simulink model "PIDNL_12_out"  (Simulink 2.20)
settings: Solver=VariableStepDiscrete  StartTime=0.0  StopTime=40.0  RelTol=1e-3  AbsTol=1e-6
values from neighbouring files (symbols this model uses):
  a = input('Inserisci il dato da graficare [1=PIDNL 2=PD 3=PID]: ')    [grp.m]    (also in grp1.m = input('Inserisci il dato da graficare [1..3]'))
undefined symbols (not defined in the file or in its folder): b, nldelta, pidin
libraries: simulink x3, Puma x2

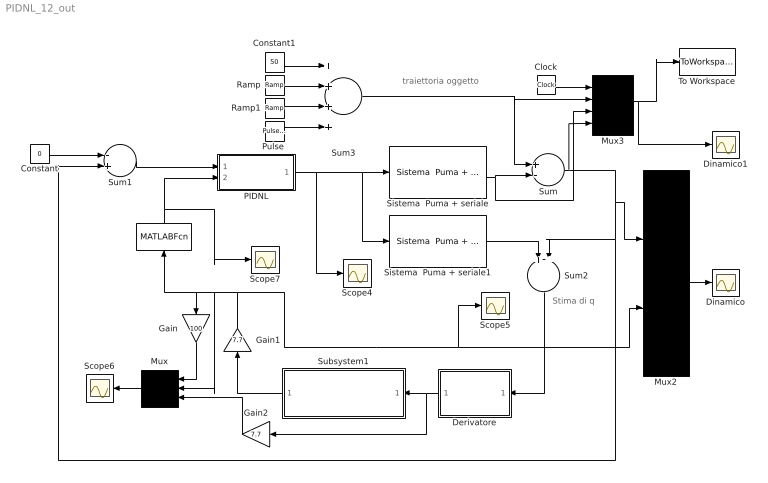
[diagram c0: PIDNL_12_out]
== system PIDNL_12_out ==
  note: Stima di q
  note: traiettoria oggetto
  " " : MATLABFcn  Orientation=up  MATLABFcn=nldelta(u(1))  OutputWidth=-1
  Clock : Clock
  Constant : Constant  Value=0
  Constant1 : Constant  Value=50
  Derivatore : Subsystem  Orientation=left  mask(Simulazione Derivatore implementato in maniera software){Td=0.13, T=0.030, N=5}
      mask prompts: Td "Costante di derivazione Td"; T "Sample Time T del PD"; N "Indice polo del derivatore [5..10]"
      mask init:
      | Kbeta=Td/(N*T+Td);
      | Kalfa=N*Kbeta;
  Dinamico : Scope
  Dinamico1 : Scope
  Gain : Gain  Orientation=down  Gain=100
  Gain1 : Gain  Orientation=up  Gain=7.7
  Gain2 : Gain  Orientation=left  Gain=7.7
  Mux : Mux  Orientation=left  Inputs=3
  Mux2 : Mux  Inputs=2
  Mux3 : Mux  Inputs=4
  PIDNL : Subsystem
  "Pulse " : simulink/Sources/Pulse Generator  period=30  duty=10  amplitude=-50  start=30
  Ramp : simulink/Sources/Ramp  slope=-50  start=10  X0=0
  Ramp1 : simulink/Sources/Ramp  slope=+50  start=25  X0=0
  Scope{4..7} (4 alike) : Scope
  Sistema  Puma + seriale : Puma/Sistema  Puma + seriale  Ts=.260
  Sistema  Puma + seriale1 : Puma/Sistema  Puma + seriale  Ts=.260
  Subsystem1 : Subsystem  Orientation=left  mask(Filtro di Butterworth){ordine=3, freq=0.1/16}
      mask prompts: ordine "Ordine del filtro"; freq "Parametro K per ricavare la Freq. di taglio Ft"
      mask help: Attenzione! Considerare il parametro Fc come la frequanza di campionamento del segnale di ingresso, per cui la frequanza di taglio diviene Ft=K*Fc;
      mask init:
      | [b,a]=butter(ordine,freq);
  Sum : Sum  Inputs=+-
  Sum1 : Sum  Inputs=-+
  Sum2 : Sum  Orientation=down  Inputs=++
  Sum3 : Sum  Inputs=++++
  To Workspace : ToWorkspace  VariableName=din  SampleTime=-1
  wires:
  Sistema  Puma + seriale1/1 -> Sum2/1
  Mux2/1 -> Dinamico/1
  Sum2/1 -> Derivatore/1(In1)
  Mux/1 -> Scope6/1
  Derivatore/1(Out1) -> Subsystem1/1(In1), Gain2/1
  Constant1/1 -> Sum3/1
  Sum1/1 -> PIDNL/1(In1)
  Constant/1 -> Sum1/1
  PIDNL/1(Out1) -> Sistema  Puma + seriale/1, Sistema  Puma + seriale1/1, Scope4/1
  Ramp/1 -> Sum3/2
  Ramp1/1 -> Sum3/3
  Subsystem1/1(Out1) -> Gain1/1
  Gain2/1 -> Mux/3
  Gain/1 -> Mux/1
  Gain1/1 -> Gain/1, " "/1, Mux/2, Scope5/1, Mux2/2
  "Pulse "/1 -> Sum3/4
  " "/1 -> PIDNL/2(In2), Scope7/1
  Mux3/1 -> To Workspace/1, Dinamico1/1
  Sistema  Puma + seriale/1 -> Sum/2, Mux3/3
  Sum3/1 -> Sum/1, Mux3/2
  Clock/1 -> Mux3/1
  Sum/1 -> Sum2/2, Sum1/2, Mux2/1, Mux3/4

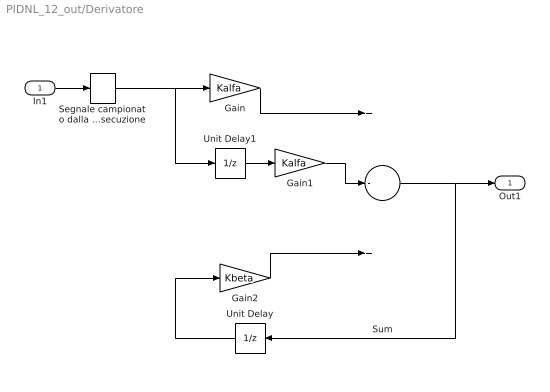
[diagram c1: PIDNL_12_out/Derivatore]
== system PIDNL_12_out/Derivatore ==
  In1 : Inport  Port=1  PortWidth=-1  SampleTime=-1
  Gain : Gain  Gain=Kalfa
  Gain1 : Gain  Gain=Kalfa
  Gain2 : Gain  Gain=Kbeta
  Segnale campionato dalla procedura software al momento del ciclo  d 'esecuzione : ZeroOrderHold  SampleTime=T
  Sum : Sum  Inputs=+-+
  Unit Delay : UnitDelay  Orientation=left  X0=0  SampleTime=T
  Unit Delay1 : UnitDelay  X0=0  SampleTime=T
  Out1 : Outport  Port=1
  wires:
  Gain1/1 -> Sum/2
  Unit Delay/1 -> Gain2/1
  Gain2/1 -> Sum/3
  Gain/1 -> Sum/1
  Unit Delay1/1 -> Gain1/1
  Sum/1 -> Out1/1, Unit Delay/1
  In1/1 -> Segnale campionato dalla procedura software al momento del ciclo  d 'esecuzione/1
  Segnale campionato dalla procedura software al momento del ciclo  d 'esecuzione/1 -> Gain/1, Unit Delay1/1

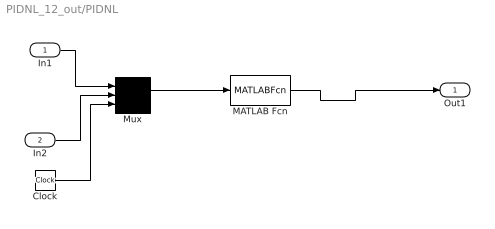
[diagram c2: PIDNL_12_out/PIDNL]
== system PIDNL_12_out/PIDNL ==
  In1 : Inport  Port=1  PortWidth=-1  SampleTime=-1
  In2 : Inport  Port=2  PortWidth=-1  SampleTime=-1
  Clock : Clock
  MATLAB Fcn : MATLABFcn  MATLABFcn=pidin(u(1),u(2),u(3))  OutputWidth=1
  Mux : Mux  Inputs=3
  Out1 : Outport  Port=1
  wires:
  MATLAB Fcn/1 -> Out1/1
  Mux/1 -> MATLAB Fcn/1
  In1/1 -> Mux/1
  In2/1 -> Mux/2
  Clock/1 -> Mux/3

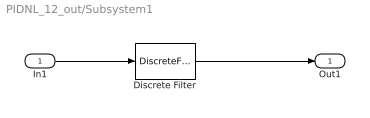
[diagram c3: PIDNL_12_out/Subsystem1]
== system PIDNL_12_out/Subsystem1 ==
  In1 : Inport  Port=1  PortWidth=-1  SampleTime=-1
  Discrete Filter : DiscreteFilter  Numerator=b  Denominator=a  SampleTime=.032
  Out1 : Outport  Port=1
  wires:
  In1/1 -> Discrete Filter/1
  Discrete Filter/1 -> Out1/1
